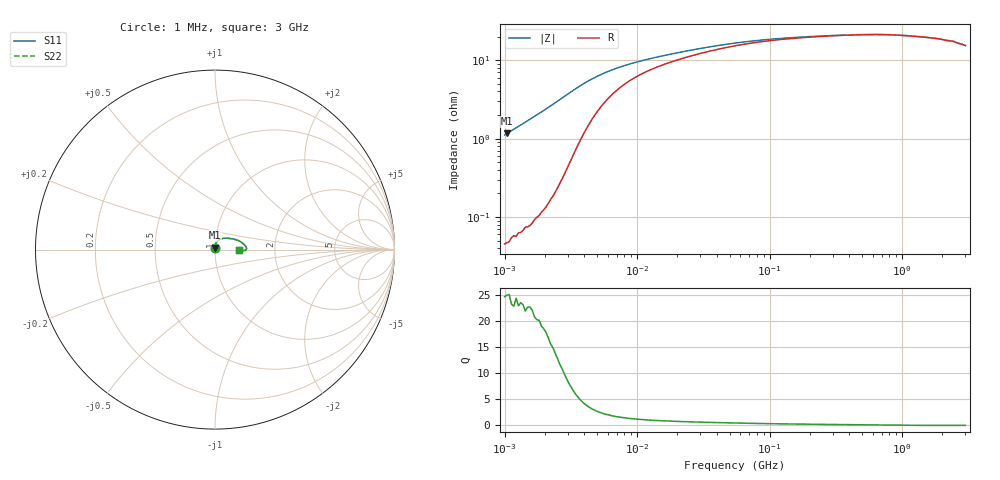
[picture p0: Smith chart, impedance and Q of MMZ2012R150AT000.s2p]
! S-parameter Generated by TDK Corporation
! Copyright(C) 2016 TDK Corporation.
! All Rights Reserved.
! TDK P/N: MMZ2012R150AT000 (Chip Beads)
! Property: |Z|=15¶ at 100MHz
! Size(LxWxT): 2x1.25x0.85mm, 0.079x0.049x0.033inches
! Model Type: s2p (Touchstone File Format Version 1.0)
! Frequency: DC=Yes Start=1MHz Stop=3000MHz 202points Log-sweep
! Note: This model was converted from impedance.
! Model Generated on May. 16, 2016
! Hash(MD5):
! Port Assignments:
!  1 ---@@@--- 2
! Applicable Conditions:
!  Temperature = 25 degC
!  DC Bias Current = 0 A
!  Small Signal Operation
! Terms and conditions regarding TDK Simulation Models
! (1)This simulation model is being provided solely for informational purposes. Please refer to the specifications of the products in terms of detailed characteristics of such products.
! (2)In no event shall TDK Corporation of any of its subsidiaries be liable for any loss or damage arising, directly or indirectly,
!  From any information contained in this simulation model, including, but not limited to loss or damages arising from any inaccuracies, omissions or errors in connection with such information.
! (3)Any and all copyrights on this simulation model are owned by TDK Corporation.
!  Duplication or redistribution of this simulation model without prior written permission from TDK Corporation is prohibited.
! (4)This simulation model is subject to any modification or change without any prior notice.
! (5)Neither TDK Corporation nor any of its subsidiaries shall make any warranty, express or implied,
!  Including but not limited to the correctness, implied warranties of merchantability and fitness for a particular purpose with respect to this simulation models.
! (6)The use of this simulation model shall be deemed to have consented to the terms and conditions hereof.
# MHz S MA R 50
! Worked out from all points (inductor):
!   201 points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, 1 MHz to 3 GHz, reference 50 ohm
!   read as one part in series: L = 179 nH near 1.041 MHz
!   highest Q = 24.6 at 1.041 MHz (marker M1), where L = 178 nH
!   self-resonance near 890.5 MHz
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1  0.01114 87.0  0.9995 -0.6  0.9995 -0.6  0.01114 87.0
1.040844  0.01164 87.0  0.9995 -0.7  0.9995 -0.7  0.01164 87.0
1.897447  0.02185 85.7  0.9986 -1.3  0.9986 -1.3  0.02185 85.7
3.32329  0.04147 78.9  0.9928 -2.3  0.9928 -2.3  0.04147 78.9
3.900413  0.04907 74.4  0.9879 -2.7  0.9879 -2.7  0.04907 74.4
4.398124  0.05496 70.4  0.983 -3.0  0.983 -3.0  0.05496 70.4
4.959344  0.06069 66.3  0.9772 -3.3  0.9772 -3.3  0.06069 66.3
5.820586  0.06802 60.8  0.9687 -3.5  0.9687 -3.5  0.06802 60.8
6.83139  0.0749 55.7  0.9597 -3.7  0.9597 -3.7  0.0749 55.7
8.017732  0.08132 50.9  0.9508 -3.8  0.9508 -3.8  0.08132 50.9
9.794439  0.08877 45.7  0.9402 -3.9  0.9402 -3.9  0.08877 45.7
14.61624  0.1025 37.3  0.9206 -3.9  0.9206 -3.9  0.1025 37.3
30.0453  0.1259 26.6  0.8892 -3.6  0.8892 -3.6  0.1259 26.6
54.77226  0.1436 19.6  0.866 -3.2  0.866 -3.2  0.1436 19.6
99.84923  0.1571 13.7  0.8481 -2.5  0.8481 -2.5  0.1571 13.7
213.6344  0.1684 8.2  0.8337 -1.6  0.8337 -1.6  0.1684 8.2
475.755  0.1754 3.6  0.825 -0.8  0.825 -0.8  0.1754 3.6
800.5644  0.1749 0.6  0.8251 -0.1  0.8251 -0.1  0.1749 0.6
1102.76  0.1708 -0.9  0.8292 0.2  0.8292 0.2  0.1708 -0.9
1782.824  0.1602 -2.0  0.8399 0.4  0.8399 0.4  0.1602 -2.0
2455.801  0.1481 -2.4  0.852 0.4  0.852 0.4  0.1481 -2.4
3000  0.1338 -1.3  0.8663 0.2  0.8663 0.2  0.1338 -1.3
